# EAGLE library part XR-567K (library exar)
TONE DECODER
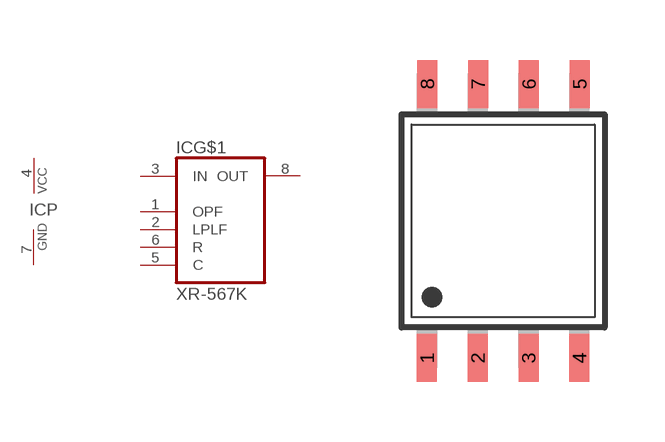
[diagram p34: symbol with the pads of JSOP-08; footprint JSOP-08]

Designator prefix IC; gates G$1=XR-567 P=PWRN

## XR-567K (OC_FARNELL: unknown; OC_NEWARK: unknown)  [JSOP-08]
1  G$1:OPF  in
2  G$1:LPLF  in
3  G$1:IN  in
4  P:VCC  pwr
5  G$1:C  in
6  G$1:R  in
7  P:GND  pwr
8  G$1:OUT  out

## Footprint JSOP-08 (pad centres in mm)
JEDEC Small Outline Package
smd 0.5 x 1.2: 1 -1.905,-3.429; 2 -0.635,-3.429; 3 0.635,-3.429; 4 1.905,-3.429; 5 1.913,3.429; 6 0.643,3.429; 7 -0.627,3.429; 8 -1.897,3.429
